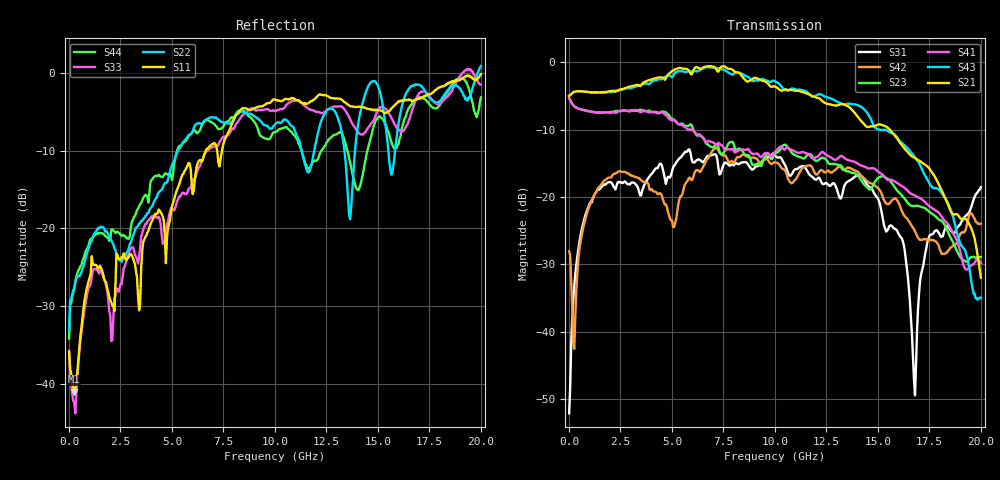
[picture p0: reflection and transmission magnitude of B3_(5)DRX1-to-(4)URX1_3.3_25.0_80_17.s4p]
!Agilent Technologies,N5225A,MY51451112,A.09.50.13
!Agilent N5225A: A.09.50.13
!Date: Sunday, March 12, 2017 05:20:51
!Correction: S11(Full 4 Port(1,2,3,4))
!S12(Full 4 Port(1,2,3,4))
!S13(Full 4 Port(1,2,3,4))
!S14(Full 4 Port(1,2,3,4))
!S21(Full 4 Port(1,2,3,4))
!S22(Full 4 Port(1,2,3,4))
!S23(Full 4 Port(1,2,3,4))
!S24(Full 4 Port(1,2,3,4))
!S31(Full 4 Port(1,2,3,4))
!S32(Full 4 Port(1,2,3,4))
!S33(Full 4 Port(1,2,3,4))
!S34(Full 4 Port(1,2,3,4))
!S41(Full 4 Port(1,2,3,4))
!S42(Full 4 Port(1,2,3,4))
!S43(Full 4 Port(1,2,3,4))
!S44(Full 4 Port(1,2,3,4))
!S4P File: Measurements: <S11,S12,S13,S14>,
!<S21,S22,S23,S24>,
!<S31,S32,S33,S34>,
!<S41,S42,S43,S44>:
# Hz S  dB  R 50
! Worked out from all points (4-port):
!   401 points, 10 MHz to 20 GHz, reference 50 ohm
!   strongest paths, dB at 10 MHz, 5.008 GHz, 10.01 GHz, 15 GHz, 20 GHz:
!     S21: -5.0, -1.3, -3.6, -9.3, -32.0
!     S43: -5.0, -2.2, -2.8, -9.9, -35.0
!     S41: -5.3, -8.7, -13.3, -16.2, -29.8
!     S23: -5.3, -8.5, -13.6, -17.2, -28.9
!     S42: -28.1, -23.5, -14.9, -18.6, -23.9
!     S31: -52.1, -16.2, -13.8, -20.2, -18.6
!   lowest |S11| = -41.0 dB at 259.9 MHz (marker M1), VSWR 1.02, Z = 50.3 - j0.859 ohm
!   |S11| at or under -10 dB: start of sweep to 6.649 GHz; 7.193 GHz to 7.433 GHz (240 MHz wide, 3.28 % of centre)
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1e7  -35.87 -38.0  -67.38 100.2  -52.40 22.0  -63.64 117.5
     -5.02 1.2  -33.23 38.5  -5.33 179.9  -27.97 37.8
     -52.09 19.1  -62.14 96.7  -35.70 -44.7  -63.19 137.7
     -5.34 179.9  -28.08 38.0  -5.00 1.3  -34.15 45.2
2.59875e8  -40.98 -73.0  -49.65 55.0  -33.21 94.5  -50.61 53.1
           -4.40 -6.8  -27.64 -131.4  -6.54 163.7  -42.00 -161.4
           -33.24 94.9  -49.98 55.7  -42.36 -79.4  -50.61 54.5
           -6.54 162.9  -42.52 -170.4  -4.39 -7.5  -27.72 -137.5
5.257375e9  -15.02 83.7  -34.86 6.0  -14.69 30.0  -34.60 -6.9
            -0.96 172.8  -10.21 140.6  -9.06 -43.8  -22.55 71.9
            -14.68 27.8  -34.79 7.5  -16.48 101.8  -36.75 7.0
            -8.98 -61.4  -22.17 69.7  -1.38 162.5  -9.97 117.8
8.30585e9  -4.88 38.0  -39.44 -99.9  -15.08 -2.0  -36.55 -139.6
           -1.71 25.7  -5.00 79.7  -12.86 -146.4  -13.83 47.6
           -15.03 -2.3  -32.61 -123.7  -5.89 57.9  -32.05 -161.4
           -13.03 -169.1  -14.07 50.2  -1.63 13.0  -4.83 44.7
1.225388e10  -2.86 -19.6  -34.78 -160.6  -17.56 -24.1  -36.38 160.0
             -5.63 -138.0  -6.15 71.2  -14.21 65.2  -15.90 37.8
             -17.81 -23.0  -34.45 -149.0  -5.20 -7.3  -33.40 164.8
             -13.38 25.5  -15.99 40.1  -4.81 -163.7  -10.07 -6.2
1.68016e10  -3.53 -76.6  -35.65 110.5  -51.22 -79.5  -36.43 83.3
            -14.23 28.7  -1.50 70.1  -21.31 -170.1  -25.23 62.8
            -49.44 -123.7  -32.94 123.0  -3.73 -83.0  -33.47 81.0
            -19.80 139.2  -25.10 63.2  -14.15 -24.1  -3.50 -60.5
2e10  -0.19 -114.0  -33.01 63.0  -18.59 121.9  -35.46 21.8
      -31.97 -109.6  0.84 17.1  -28.90 49.5  -23.92 102.0
      -18.56 121.8  -33.97 40.0  -1.54 -87.6  -35.20 -7.8
      -29.79 10.1  -23.95 102.7  -34.97 -136.6  -3.17 -136.4
